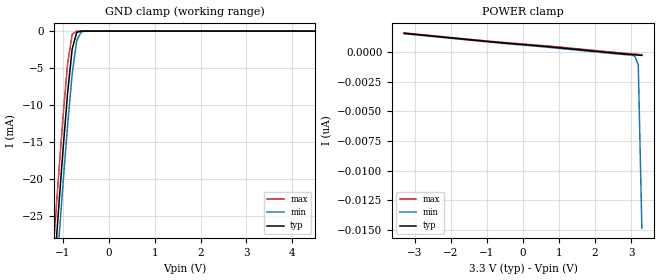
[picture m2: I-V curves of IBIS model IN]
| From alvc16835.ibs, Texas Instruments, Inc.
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|   Model ALVC16835_IN
[Model]   IN
Model_type   Input
Polarity   Non-Inverting
Vinl = 0.8V
Vinh = 2.0V
|Variable   typ   min   max
C_comp   6pF   NA   NA
[Voltage Range]   3.3   3.0   3.6
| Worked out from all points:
|   GND clamp passes 1 mA (typ) near -0.74 V on its own axis
[POWER_Clamp]   | Note: Vtable = Vcc - Voutput
|   Voltage   I(typ)   I(min)   I(max)
-3.3V     1.569nA    1.535nA    1.605nA
3.1V      -240.8pA   -336.6pA   -183.8pA
3.2V      -265.7pA   -1.088nA   -208.7pA
3.3V      -290.6pA   -14.86nA   -233.6pA
[GND_Clamp]
|   Voltage   I(typ)   I(min)   I(max)
-3.3V     -226.9mA   -231.1mA   -222.8mA
-1.2V     -33.05mA   -37.73mA   -28.48mA
-1.1V     -24.41mA   -29.09mA   -19.85mA
-1V       -16.09mA   -20.7mA    -11.63mA
-900mV    -8.415mA   -12.77mA   -4.423mA
-800mV    -2.415mA   -5.819mA   -431.6uA
-700mV    -180.1uA   -1.262mA   -9.285uA
-600mV    -6.421uA   -95.7uA    -168.1nA
-500mV    -216nA     -5.197uA   -3.449nA
6.6V      1.569nA    1.625nA    1.515nA
